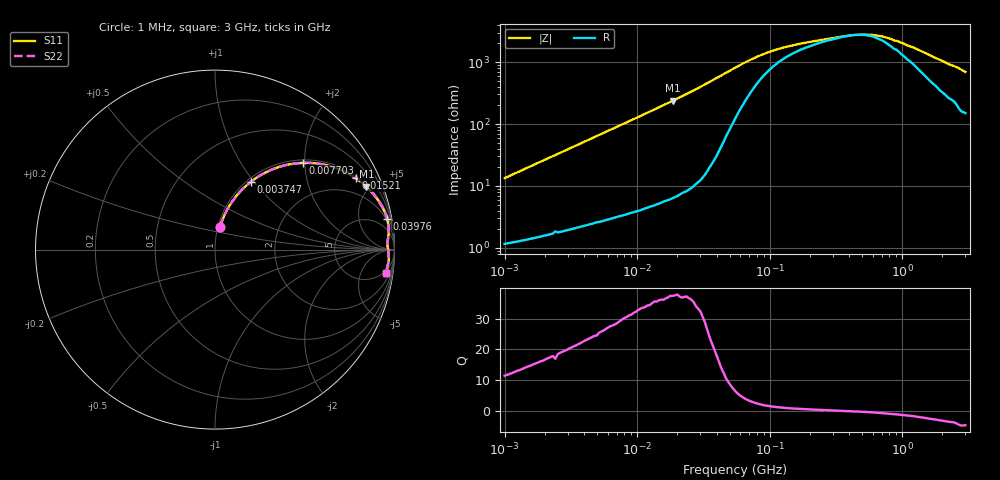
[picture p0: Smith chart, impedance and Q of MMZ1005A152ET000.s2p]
! S-parameter Generated by TDK Corporation
! Copyright(C) 2016 TDK Corporation.
! All Rights Reserved.
! TDK P/N: MMZ1005A152ET000 (Chip Beads)
! Property: |Z|=1500¶ at 100MHz
! Size(LxWxT): 1x0.5x0.5mm, 0.039x0.02x0.02inches
! Model Type: s2p (Touchstone File Format Version 1.0)
! Frequency: DC=Yes Start=1MHz Stop=3000MHz 202points Log-sweep
! Note: This model was converted from impedance.
! Model Generated on May. 16, 2016
! Hash(MD5):
! Port Assignments:
!  1 ---@@@--- 2
! Applicable Conditions:
!  Temperature = 25 degC
!  DC Bias Current = 0 A
!  Small Signal Operation
! Terms and conditions regarding TDK Simulation Models
! (1)This simulation model is being provided solely for informational purposes. Please refer to the specifications of the products in terms of detailed characteristics of such products.
! (2)In no event shall TDK Corporation of any of its subsidiaries be liable for any loss or damage arising, directly or indirectly,
!  From any information contained in this simulation model, including, but not limited to loss or damages arising from any inaccuracies, omissions or errors in connection with such information.
! (3)Any and all copyrights on this simulation model are owned by TDK Corporation.
!  Duplication or redistribution of this simulation model without prior written permission from TDK Corporation is prohibited.
! (4)This simulation model is subject to any modification or change without any prior notice.
! (5)Neither TDK Corporation nor any of its subsidiaries shall make any warranty, express or implied,
!  Including but not limited to the correctness, implied warranties of merchantability and fitness for a particular purpose with respect to this simulation models.
! (6)The use of this simulation model shall be deemed to have consented to the terms and conditions hereof.
# MHz S MA R 50
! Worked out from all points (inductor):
!   201 points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, 1 MHz to 3 GHz, reference 50 ohm
!   read as one part in series: L = 2.11 uH near 1.041 MHz
!   highest Q = 37.4 at 18.58 MHz (marker M1), where L = 2.04 uH
!   self-resonance near 433.8 MHz
!   S11 on the Smith chart (normalised r, x): 1 MHz: 1.02, +0.27; 3.747 MHz: 1.04, +0.97; 7.703 MHz: 1.07, +1.96; 15.21 MHz: 1.11, +3.87; 39.76 MHz: 2, +11; 3 GHz: 4, -14
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1  0.1308 77.5  0.9801 -7.5  0.9801 -7.5  0.1308 77.5
2.13957  0.2664 71.3  0.9485 -15.4  0.9485 -15.4  0.2664 71.3
3.747356  0.4287 62.0  0.8842 -25.4  0.8842 -25.4  0.4287 62.0
3.900413  0.4424 61.2  0.8774 -26.2  0.8774 -26.2  0.4424 61.2
5.592179  0.5726 52.9  0.7982 -34.9  0.7982 -34.9  0.5726 52.9
7.703107  0.6895 44.5  0.7015 -43.6  0.7015 -43.6  0.6895 44.5
10.61086  0.7921 35.9  0.587 -52.4  0.587 -52.4  0.7921 35.9
14.61624  0.8708 27.9  0.468 -60.5  0.468 -60.5  0.8708 27.9
15.21322  0.8788 27.0  0.4535 -61.5  0.4535 -61.5  0.8788 27.0
18.58443  0.9132 22.6  0.3839 -65.9  0.3839 -65.9  0.9132 22.6
26.64524  0.9541 15.9  0.2738 -72.5  0.2738 -72.5  0.9541 15.9
39.76269  0.9747 10.1  0.176 -76.7  0.176 -76.7  0.9747 10.1
54.77226  0.9751 6.8  0.1201 -74.6  0.1201 -74.6  0.9751 6.8
81.73662  0.9678 4.1  0.07789 -63.5  0.07789 -63.5  0.9678 4.1
103.9275  0.9641 3.1  0.06384 -54.2  0.06384 -54.2  0.9641 3.1
149.005  0.9614 2.0  0.05149 -40.5  0.05149 -40.5  0.9614 2.0
213.6344  0.9611 1.2  0.04431 -27.9  0.04431 -27.9  0.9611 1.2
495.1867  0.9657 -0.3  0.03455 7.3  0.03455 7.3  0.9657 -0.3
581.181  0.9668 -0.6  0.03476 16.9  0.03476 16.9  0.9668 -0.6
800.5644  0.9685 -1.5  0.04022 37.7  0.04022 37.7  0.9685 -1.5
1243.477  0.9689 -2.8  0.05738 55.8  0.05738 55.8  0.9689 -2.8
3000  0.9608 -7.8  0.1384 69.7  0.1384 69.7  0.9608 -7.8
